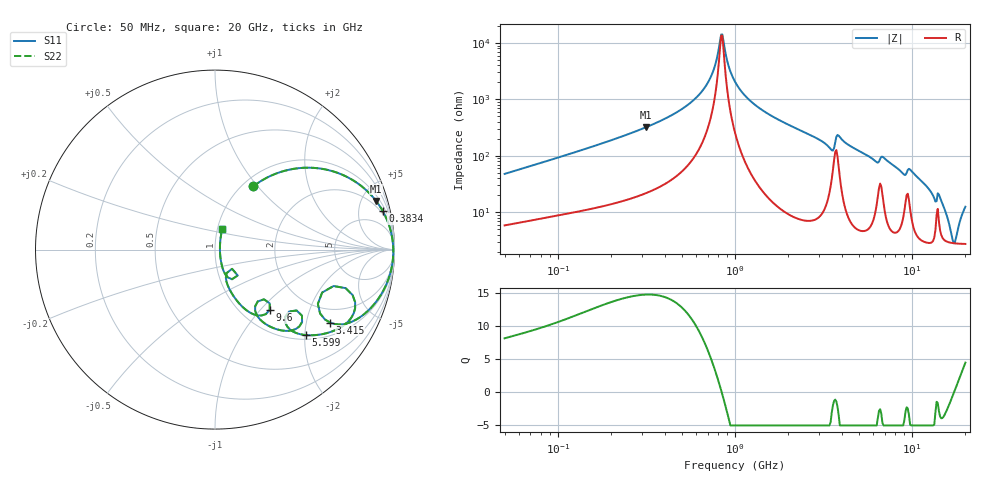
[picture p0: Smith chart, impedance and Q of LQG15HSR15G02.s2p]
!Murata Part Number: LQG15HSR15G02
!These Parameters are Measured in Series Mode Connection
!  o--[Z]--o
!Port1  Port2
!  o-------o
!Freq. Start=50[MHz] Stop=20[GHz], 401[Steps]
# Hz S RI R 50
!Freq.(Hz) S11(Real) S11(Imag) S21(Real) S21(Imag) S12(Real) S12(Imag) S22(Real) S22(Imag)
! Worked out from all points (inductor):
!   401 points, 50 MHz to 20 GHz, reference 50 ohm
!   read as one part in series: L = 149 nH near 51.52 MHz
!   highest Q = 14.7 at 315.6 MHz (marker M1), where L = 162 nH
!   self-resonance near 835.5 MHz
!   S11 on the Smith chart (normalised r, x): 50 MHz: 1.12, +0.95; 383.4 MHz: 1.58, +8.44; 3.415 GHz: 1.44, -2.76; 5.599 GHz: 1.10, -2.02; 9.6 GHz: 1.33, -1.13; 20 GHz: 1.05, +0.24
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5e7  0.2134 0.3527  0.7866 -0.3527  0.7866 -0.3527  0.2134 0.3527
1.364002e8  0.6072 0.4482  0.3928 -0.4482  0.3928 -0.4482  0.6072 0.4482
3.155756e8  0.8972 0.2716  0.1028 -0.2716  0.1028 -0.2716  0.8972 0.2716
3.721004e8  0.9288 0.2251  0.0712 -0.2251  0.0712 -0.2251  0.9288 0.2251
3.834161e8  0.9337 0.2167  0.0663 -0.2167  0.0663 -0.2167  0.9337 0.2167
6.574395e8  0.987 0.067  0.013 -0.067  0.013 -0.067  0.987 0.067
7.523192e8  0.9917 0.0304  0.00831 -0.0304  0.00831 -0.0304  0.9917 0.0304
8.354841e8  0.9932 0.0019  0.00675 -0.0019  0.00675 -0.0019  0.9932 0.0019
1e9  0.9917 -0.0474  0.00828 0.0474  0.00828 0.0474  0.9917 -0.0474
1.411297e9  0.9723 -0.1464  0.0277 0.1464  0.0277 0.1464  0.9723 -0.1464
2.728004e9  0.8275 -0.3623  0.1725 0.3623  0.1725 0.3623  0.8275 -0.3623
3.415248e9  0.6399 -0.4062  0.3601 0.4062  0.3601 0.4062  0.6399 -0.4062
3.792786e9  0.7666 -0.2528  0.2334 0.2528  0.2334 0.2528  0.7666 -0.2528
4.275624e9  0.7173 -0.4221  0.2827 0.4221  0.2827 0.4221  0.7173 -0.4221
5.598765e9  0.5057 -0.4763  0.4943 0.4763  0.4943 0.4763  0.5057 -0.4763
6.503449e9  0.4131 -0.3444  0.5869 0.3444  0.5869 0.3444  0.4131 -0.3444
7.442007e9  0.3772 -0.4513  0.6228 0.4513  0.6228 0.4513  0.3772 -0.4513
8.774992e9  0.2312 -0.3618  0.7688 0.3618  0.7688 0.3618  0.2312 -0.3618
9.600142e9  0.3048 -0.3367  0.6952 0.3367  0.6952 0.3367  0.3048 -0.3367
1.438523e10  0.0719 -0.155  0.9281 0.155  0.9281 0.155  0.0719 -0.155
1.721783e10  0.0274 -0.00204  0.9726 0.00204  0.9726 0.00204  0.0274 -0.00204
2e10  0.0403 0.1143  0.9597 -0.1143  0.9597 -0.1143  0.0403 0.1143
